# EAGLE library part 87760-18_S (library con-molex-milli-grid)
HEADER
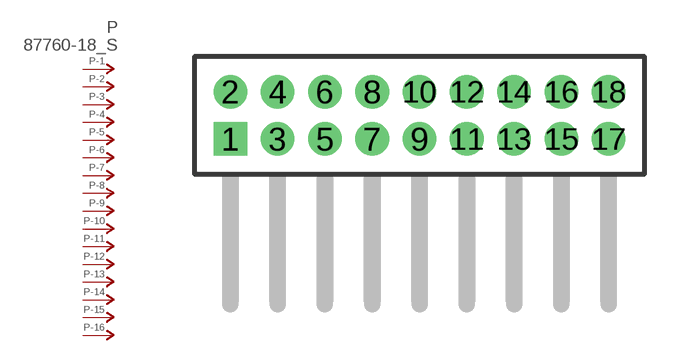
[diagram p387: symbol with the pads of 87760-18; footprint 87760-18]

Designator prefix P; gates -1=P-NV -2=P-N -3=P-N -4=P-N -5=P-N -6=P-N -7=P-N -8=P-N -9=P-N -10=P-N -11=P-N -12=P-N -13=P-N -14=P-N -15=P-N -16=P-N -17=P-N -18=P-N

## 87760-18_S  [87760-18]
1  -1:P  pas
2  -2:P  pas
3  -3:P  pas
4  -4:P  pas
5  -5:P  pas
6  -6:P  pas
7  -7:P  pas
8  -8:P  pas
9  -9:P  pas
10  -10:P  pas
11  -11:P  pas
12  -12:P  pas
13  -13:P  pas
14  -14:P  pas
15  -15:P  pas
16  -16:P  pas
17  -17:P  pas
18  -18:P  pas

## Footprint 87760-18 (pad centres in mm)
HEADER Dual Row, Right Angle
drill 0.914 square: 1 -8,-1
drill 0.914: 2 -8,1; 3 -6,-1; 4 -6,1; 5 -4,-1; 6 -4,1; 7 -2,-1; 8 -2,1; 9 0,-1; 10 0,1; 11 2,-1; 12 2,1; 13 4,-1; 14 4,1; 15 6,-1; 16 6,1; 17 8,-1; 18 8,1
